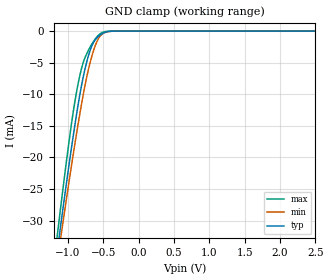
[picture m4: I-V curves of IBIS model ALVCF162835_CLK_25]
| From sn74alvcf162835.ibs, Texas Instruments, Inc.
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[Model]   ALVCF162835_CLK_25
Model_type  Input
Vinl=0.7
Vinh=1.7
| variable   typ   min   max
C_comp   2.47pF   2.05pF   3.00pF
[Temperature Range]   40   100   -40
| Ambient temperature   25   85   -40
[Voltage range]   2.5   2.3   2.7
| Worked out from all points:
|   GND clamp passes 1 mA (typ) near -0.58 V on its own axis
[GND Clamp]
| ALVCF162835_CLK_25
|   Voltage   I(typ)   I(min)   I(max)
-2.5V     -157.4mA   -149.3mA   -167.1mA
-1.145V   -34.29mA   -36.03mA   -31.77mA
-1.105V   -30.94mA   -32.93mA   -28.09mA
-1.085V   -29.29mA   -31.39mA   -26.27mA
-930mV    -16.95mA   -19.85mA   -13.14mA
-820mV    -9.331mA   -12.32mA   -6.453mA
-745mV    -5.343mA   -7.848mA   -3.848mA
-675mV    -2.707mA   -4.493mA   -2.304mA
-595mV    -1.137mA   -1.781mA   -967.5uA
-525mV    -460.4uA   -560.8uA   -284.1uA
-340mV    -6.934uA   -11.03uA   -976nA
2.5V      156.4pA    885pA      34.32pA
